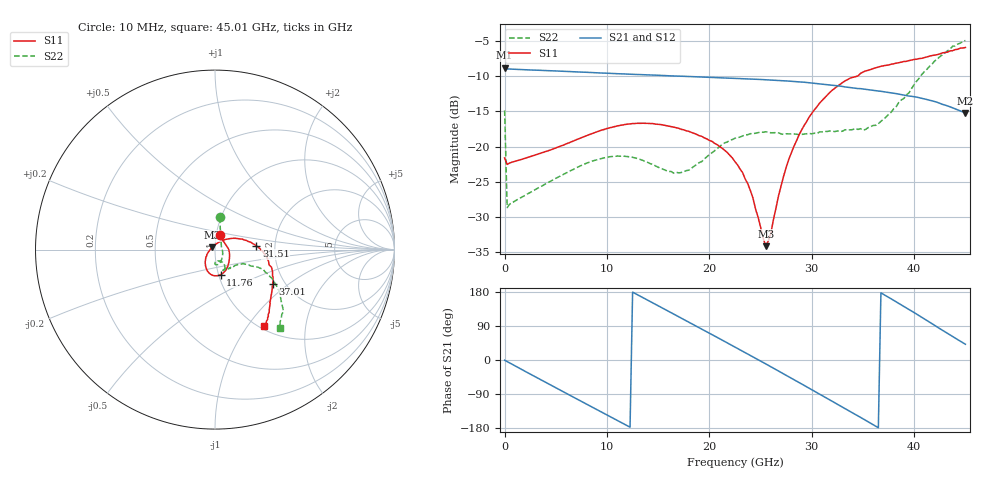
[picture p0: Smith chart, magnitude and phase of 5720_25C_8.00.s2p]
! Device:  ADRF5720
! Description: 0.5dB LSB GaAs MMIC 6-bit Digital Attenuator
! Frequency:  0.000009 -  40 GHz
! Ports:
!	RF1	= Port 1
!	RF2	= Port 2
! Vdd:  3.3 Volt
! Vss:  -3.3 Volt
! Control:  0/3.3 Volt
! State:  8.00 dB attenuation
! Data:  The device was measured using G-S-G Probes on a matrix board.
!  Data was collected using an calibrated 4 port network analyzer.
!  The reference plane for this measurement is at the launchers.
! Note:  Analog Devices supplies this data as a sample of measured data
!  for this product.  Your particular data for this product may vary.
!  Data was taken at 25 degrees C.
!  Analog Devices reserves the right to change this data at anytime.
# GHZ S DB R 45.0
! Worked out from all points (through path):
!   181 points, 10 MHz to 45.01 GHz, reference 45 ohm
!   highest |S21| = -8.80 dB at 10 MHz (marker M1); lowest = -15.2 dB at 45.01 GHz (marker M2)
!   group delay of S21, straight-line fit = 41.5 ps
!   lowest |S11| = -34.1 dB at 25.51 GHz (marker M3), VSWR 1.04, Z = 43.6 + j1.07 ohm
!   |S11| at or under -10 dB: start of sweep to 34.46 GHz
!   |S22| runs from -28.7 to -4.9 dB; largest |S21 - S12| = 0.00045
!   S11 on the Smith chart (normalised r, x): 10 MHz: 1.04, +0.17; 11.76 GHz: 1.02, -0.29; 31.51 GHz: 1.60, +0.07; 37.01 GHz: 1.74, -0.77; 45.01 GHz: 1.06, -1.20
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0.01  -21.63 72.1  -8.80 -0.6  -8.80 -0.6  -14.86 81.8
0.26  -22.54 4.4  -8.98 -4.1  -8.98 -4.1  -28.67 9.8
4.26  -20.60 -30.4  -9.23 -62.5  -9.23 -62.4  -25.10 -42.0
7.76  -18.60 -52.7  -9.45 -112.8  -9.45 -112.8  -22.52 -65.2
11.76  -16.88 -77.3  -9.70 -170.2  -9.71 -170.1  -21.39 -85.0
15.26  -16.88 -96.3  -9.90 139.5  -9.90 139.5  -23.09 -88.4
17.01  -17.41 -104.4  -10.00 114.2  -10.01 114.3  -23.75 -76.9
19.01  -18.46 -112.8  -10.12 85.2  -10.12 85.2  -22.29 -61.6
22.76  -22.61 -135.3  -10.34 30.5  -10.35 30.5  -18.75 -61.1
24.26  -27.29 -156.3  -10.44 8.4  -10.45 8.4  -18.16 -64.8
25.51  -34.15 141.1  -10.51 -10.2  -10.52 -10.2  -17.91 -67.8
26.01  -32.33 96.8  -10.55 -17.7  -10.55 -17.7  -18.05 -68.0
26.76  -27.00 64.7  -10.61 -29.0  -10.61 -29.0  -18.06 -67.4
27.76  -21.83 44.7  -10.71 -44.2  -10.71 -44.1  -18.21 -67.0
30.26  -14.78 16.2  -11.02 -82.4  -11.02 -82.3  -18.11 -62.4
31.51  -12.73 5.1  -11.23 -101.5  -11.24 -101.4  -17.87 -59.5
34.76  -9.63 -17.3  -11.78 -151.2  -11.79 -151.2  -17.46 -49.8
37.01  -8.54 -30.5  -12.22 173.3  -12.22 173.4  -16.14 -31.5
37.76  -8.31 -33.7  -12.38 161.5  -12.38 161.5  -15.14 -26.6
41.26  -7.28 -44.8  -13.33 104.0  -13.33 104.1  -9.02 -26.7
43.76  -6.39 -52.3  -14.50 62.0  -14.50 62.0  -5.76 -42.2
45.01  -5.94 -57.0  -15.24 41.6  -15.24 41.7  -4.94 -50.5
